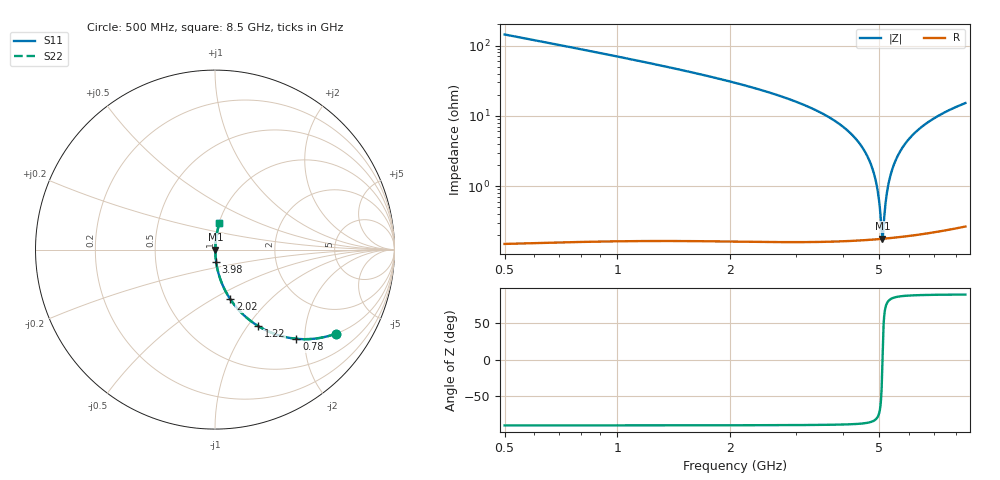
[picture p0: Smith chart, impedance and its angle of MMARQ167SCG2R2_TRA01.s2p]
! MMARQ167SCG2R2_TRA01  S-PARAMETER MODEL  ( General Type )
! Model Generated by TAIYO YUDEN Corporation (http://www.ty-top.com)
! Version 1.0
! TAIYO YUDEN Control No. 150305
! Copyright(c) 2015 TAIYO YUDEN CO.,LTD. All Rights Reserved.
! Product Description (link to TY-COMPAS)
! https://ds.yuden.co.jp/TYCOMPAS/or/detail?pn=MMARQ167SCG2R2BTRA01&u=M
! Products Name : Multilayer Ceramic Capacitors
! Characteristics :
!  Capacitance : 2.2 pF , Rated Voltage : 250V , TCC : CG / C0G
!  Case Size : 1.6 x 0.8 / 0.063 x 0.031 [mm/inch] , Thickness : 0.7 / 0.028 [mm/inch]
!  (Conditions: Temperature = 25 degC , DC Bias Current/Voltage = 0A / 0V)
! External Node Assignments :
!  1  o---| |---o  2
! GND o---------o GND
! Frequency Range : 500MHz  -  8.5GHz  [ 401 STEP ]
# MHz S RI R 50
! Freq[MHz].  S11 Real  S11 Imag  S21 Real  S21 Imag  S12 Real  S12 Imag  S22 Real  S22 Imag
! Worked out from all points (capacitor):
!   401 points, 500 MHz to 8.5 GHz, reference 50 ohm
!   read as one part in series: C = 2.19 pF near 540 MHz
!   lowest |Z| = 179 mohm at 5.1 GHz (marker M1)
!   series resonance near 5.104 GHz, so ESL is about 440 pH
!   S11 on the Smith chart (normalised r, x): 500 MHz: 1.00, -2.88; 780 MHz: 1.00, -1.82; 1.22 GHz: 1.00, -1.12; 2.02 GHz: 1.00, -0.61; 3.98 GHz: 1.00, -0.14; 8.5 GHz: 1.01, +0.30
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500  0.6747 -0.468  0.3253 0.468  0.3253 0.468  0.6747 -0.468
780  0.4534 -0.497  0.5466 0.497  0.5466 0.497  0.4534 -0.497
1220  0.2408 -0.4261  0.7592 0.4261  0.7592 0.4261  0.2408 -0.4261
1840  0.107 -0.3067  0.893 0.3067  0.893 0.3067  0.107 -0.3067
2020  0.0857 -0.2773  0.9143 0.2773  0.9143 0.2773  0.0857 -0.2773
3180  0.0207 -0.137  0.9793 0.137  0.9793 0.137  0.0207 -0.137
3980  0.00672 -0.0711  0.9933 0.0711  0.9933 0.0711  0.00672 -0.0711
4500  0.00297 -0.0359  0.997 0.0359  0.997 0.0359  0.00297 -0.0359
4720  0.00221 -0.0223  0.9978 0.0223  0.9978 0.0223  0.00221 -0.0223
4880  0.0019 -0.0128  0.9981 0.0128  0.9981 0.0128  0.0019 -0.0128
4980  0.0018 -0.00702  0.9982 0.00702  0.9982 0.00702  0.0018 -0.00702
5080  0.00176 -0.00137  0.9982 0.00137  0.9982 0.00137  0.00176 -0.00137
5100  0.00177 -0.000249  0.9982 0.000249  0.9982 0.000249  0.00177 -0.000249
5140  0.00178 0.00197  0.9982 -0.00197  0.9982 -0.00197  0.00178 0.00197
5200  0.00181 0.00527  0.9982 -0.00527  0.9982 -0.00527  0.00181 0.00527
5240  0.00184 0.00745  0.9982 -0.00745  0.9982 -0.00745  0.00184 0.00745
5360  0.002 0.0139  0.998 -0.0139  0.998 -0.0139  0.002 0.0139
5560  0.00244 0.0243  0.9976 -0.0243  0.9976 -0.0243  0.00244 0.0243
5840  0.00338 0.0383  0.9966 -0.0383  0.9966 -0.0383  0.00338 0.0383
6400  0.00622 0.0646  0.9938 -0.0646  0.9938 -0.0646  0.00622 0.0646
7180  0.0119 0.0979  0.9881 -0.0979  0.9881 -0.0979  0.0119 0.0979
8500  0.025 0.1477  0.975 -0.1477  0.975 -0.1477  0.025 0.1477
